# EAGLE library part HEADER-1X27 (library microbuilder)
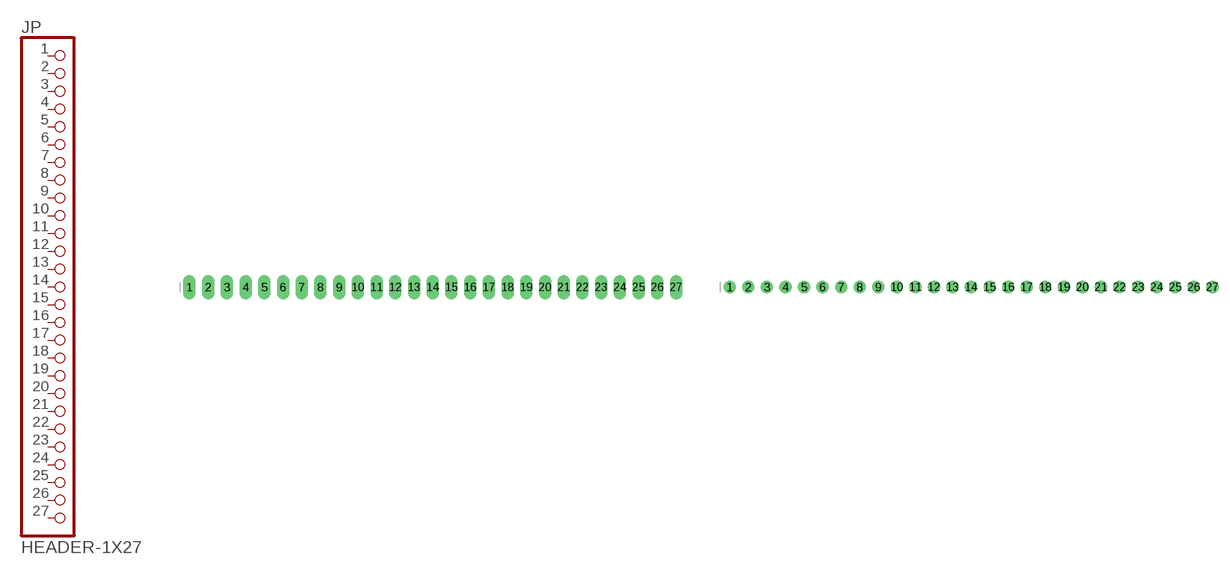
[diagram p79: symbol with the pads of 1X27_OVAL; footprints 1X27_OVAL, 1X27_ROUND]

Designator prefix JP

## HEADER-1X27  [1X27_OVAL]
1  1  pas
2  2  pas
3  3  pas
4  4  pas
5  5  pas
6  6  pas
7  7  pas
8  8  pas
9  9  pas
10  10  pas
11  11  pas
12  12  pas
13  13  pas
14  14  pas
15  15  pas
16  16  pas
17  17  pas
18  18  pas
19  19  pas
20  20  pas
21  21  pas
22  22  pas
23  23  pas
24  24  pas
25  25  pas
26  26  pas
27  27  pas

## HEADER-1X27ROUND  [1X27_ROUND]
Pads as for 1X27_OVAL

## Footprint 1X27_OVAL (pad centres in mm)
drill 1 pad 1.676 long: 1 -34.29,0; 2 -31.75,0; 3 -29.21,0; 4 -26.67,0; 5 -24.13,0; 6 -21.59,0; 7 -19.05,0; 8 -16.51,0; 9 -13.97,0; 10 -11.43,0; 11 -8.89,0; 12 -6.35,0; 13 -3.81,0; 14 -1.27,0; 15 1.27,0; 16 3.81,0; 17 6.35,0; 18 8.89,0; 19 11.43,0; 20 13.97,0; 21 16.51,0; 22 19.05,0; 23 21.59,0; 24 24.13,0; 25 26.67,0; 26 29.21,0; 27 31.75,0

## Footprint 1X27_ROUND (pad centres in mm)
drill 1 pad 1.676: 1 -33.02,0; 2 -30.48,0; 3 -27.94,0; 4 -25.4,0; 5 -22.86,0; 6 -20.32,0; 7 -17.78,0; 8 -15.24,0; 9 -12.7,0; 10 -10.16,0; 11 -7.62,0; 12 -5.08,0; 13 -2.54,0; 14 0,0; 15 2.54,0; 16 5.08,0; 17 7.62,0; 18 10.16,0; 19 12.7,0; 20 15.24,0; 21 17.78,0; 22 20.32,0; 23 22.86,0; 24 25.4,0; 25 27.94,0; 26 30.48,0; 27 33.02,0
